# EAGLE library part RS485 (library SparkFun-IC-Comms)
RS-485 Transceiver SP3485 Series 8 Pin NSOIC 3.3 V Low Power Half Duplex RS-485 Transceiver MAX3485 compatible Datasheet SparkFun Products SparkFun Transceiver Breakout - RS-485 (BOB-10124) SparkFun USB to RS-485 Converter (BOB-09822)
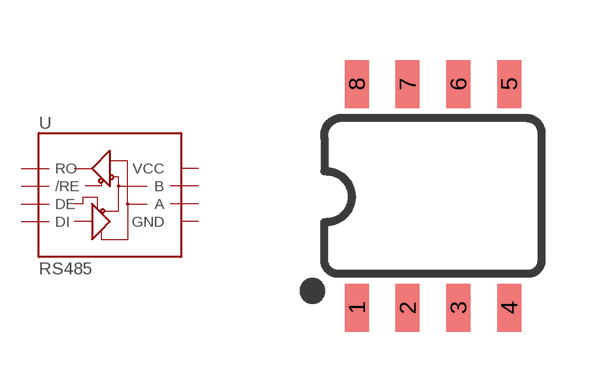
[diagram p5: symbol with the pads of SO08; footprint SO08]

Designator prefix U

## RS485SOIC (PROD_ID: IC-09388; VALUE: MAX3485CSA)  [SO08]
1  RO
2  /RE
3  DE
4  DI
5  GND
6  A
7  B
8  VCC

## Footprint SO08 (pad centres in mm)
SOIC -8 Specifications: Pin count: 8 Width: 0.15" Example device(s): MCP2551
smd 0.6 x 1.2: 1 -1.905,-2.8; 2 -0.635,-2.8; 3 0.635,-2.8; 4 1.905,-2.8; 5 1.905,2.8; 6 0.635,2.8; 7 -0.635,2.8; 8 -1.905,2.8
